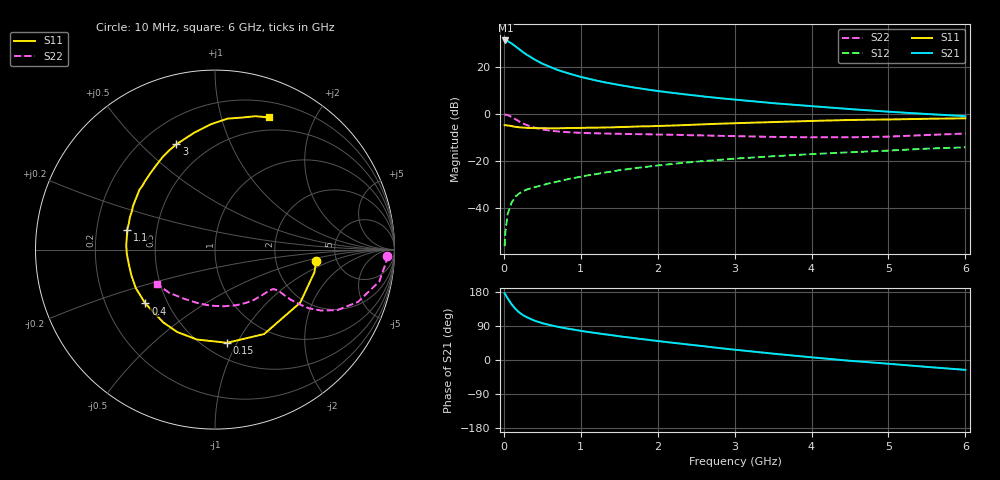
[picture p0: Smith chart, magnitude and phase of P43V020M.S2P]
! SIEMENS Small Signal Semiconductors
! BFP182
! Si NPN RF Bipolar Junction Transistor in SOT143
! VCE = 3 V  IC = 20 mA
! Common Emitter S-Parameters:  March  1996
# GHz  S  MA  R  50
!  f  S11  S21  S12  S22
! GHz  MAG  ANG  MAG  ANG  MAG  ANG  MAG  ANG
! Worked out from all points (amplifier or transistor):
!   36 points, 10 MHz to 6 GHz, reference 50 ohm
!   highest |S21| = 31.2 dB at 20 MHz (marker M1)
!   |S21| within 3 dB of that: start of sweep to 171.1 MHz
!   unconditionally stable (mu >= 1): 725.8 MHz to 5.334 GHz
!   at 250 MHz: K = 0.51, MSG = 29.6 dB, |S12| = -33.1 dB
!   at 1.4 GHz: K = 1.18, MAG = 16.2 dB, |S12| = -24.7 dB
!   at 6 GHz: K = 0.93, MSG = 6.6 dB, |S12| = -14.4 dB
!   S11 on the Smith chart (normalised r, x): 10 MHz: 3.49, -0.66; 150 MHz: 0.64, -0.91; 400 MHz: 0.38, -0.30; 1.1 GHz: 0.34, +0.10; 3 GHz: 0.33, +0.64; 6 GHz: 0.36, +1.43
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0.01  0.5682 -6.5  36.22 176.3  0.0015 79.0  0.9606 -2.0
0.02  0.5677 -13.0  36.25 173.1  0.003 84.8  0.9554 -4.3
0.05  0.5593 -31.9  35.13 162.4  0.0073 77.6  0.9323 -11.0
0.1  0.5444 -59.8  31.3 147.2  0.0127 65.1  0.8481 -20.1
0.15  0.5235 -82.6  27.27 135.0  0.017 58.6  0.7608 -26.3
0.2  0.511 -101.3  23.61 125.4  0.02 55.6  0.6813 -29.9
0.25  0.5052 -114.5  20.39 118.3  0.0222 52.7  0.6172 -32.0
0.3  0.4977 -125.3  17.93 112.7  0.0242 52.0  0.5687 -32.8
0.4  0.4906 -142.3  14.22 103.7  0.0271 50.1  0.5024 -33.5
0.5  0.4907 -154.1  11.62 97.2  0.0299 49.6  0.4606 -33.3
0.6  0.4875 -163.0  9.916 92.1  0.033 51.7  0.4353 -33.1
0.7  0.4872 -170.7  8.521 87.7  0.0357 52.2  0.4181 -33.2
0.9  0.4953 177.3  6.751 80.5  0.0422 52.9  0.3964 -33.8
1.1  0.5017 167.4  5.554 73.8  0.0487 54.1  0.3849 -35.5
1.5  0.5172 152.1  4.077 62.6  0.0623 53.4  0.3721 -40.1
1.8  0.5373 141.6  3.391 55.0  0.0718 52.4  0.3646 -44.8
2.2  0.5581 130.0  2.76 45.4  0.085 49.7  0.3552 -51.9
3  0.6247 110.2  1.994 27.2  0.11 43.1  0.3321 -69.0
3.5  0.6615 100.1  1.674 16.8  0.1236 38.8  0.3193 -81.6
4.5  0.7332 84.5  1.251 -2.1  0.1505 30.3  0.3135 -109.3
5.5  0.7767 73.1  0.982 -18.2  0.1797 22.1  0.3507 -136.6
6  0.7953 67.8  0.883 -26.0  0.1915 17.0  0.3762 -149.4
